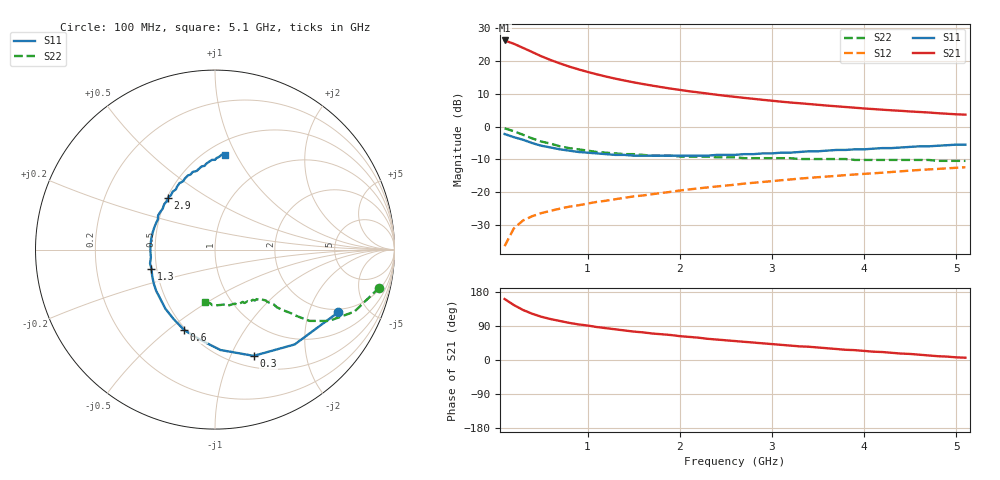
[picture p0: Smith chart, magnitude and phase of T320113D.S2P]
!AT-32011
!S PARAMETERS at Vce=2.7 V  Ic=7.5mA.  LAST UPDATED 01-05-95
# ghz s ma r 50
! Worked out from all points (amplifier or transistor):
!   51 points, 100 MHz to 5.1 GHz, reference 50 ohm
!   highest |S21| = 26.3 dB at 100 MHz (marker M1)
!   |S21| within 3 dB of that: start of sweep to 357.8 MHz
!   unconditionally stable (mu >= 1): 1.554 GHz to 4.921 GHz
!   at 900 MHz: K = 0.79, MSG = 20.7 dB, |S12| = -24.0 dB
!   at 2.6 GHz: K = 1.10, MAG = 11.5 dB, |S12| = -17.7 dB
!   at 5.1 GHz: K = 0.99, MSG = 8.0 dB, |S12| = -12.4 dB
!   S11 on the Smith chart (normalised r, x): 100 MHz: 1.84, -3.17; 300 MHz: 0.62, -1.23; 600 MHz: 0.49, -0.57; 1.3 GHz: 0.47, -0.12; 2.9 GHz: 0.51, +0.35; 5.1 GHz: 0.61, +0.90
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0.1  0.77 -27.0  20.59 161.0  0.015 76.0  0.94 -13.0
0.2  0.69 -50.0  18.33 145.0  0.028 67.0  0.85 -24.0
0.3  0.63 -70.0  15.87 132.0  0.037 60.0  0.75 -32.0
0.4  0.56 -87.0  13.7 122.0  0.043 55.0  0.66 -37.0
0.5  0.51 -99.0  11.8 114.0  0.048 53.0  0.59 -39.0
0.6  0.48 -111.0  10.35 108.0  0.052 52.0  0.55 -40.0
0.7  0.45 -121.0  9.2 103.0  0.056 51.0  0.5 -42.0
0.8  0.43 -130.0  8.24 98.0  0.06 51.0  0.47 -43.0
0.9  0.41 -138.0  7.47 94.0  0.063 51.0  0.45 -43.0
1  0.4 -145.0  6.82 91.0  0.067 51.0  0.43 -44.0
1.1  0.39 -151.0  6.27 87.0  0.071 51.0  0.41 -45.0
1.3  0.37 -163.0  5.39 81.0  0.078 52.0  0.39 -46.0
1.5  0.36 -173.0  4.73 75.0  0.086 52.0  0.38 -48.0
1.8  0.36 173.0  4 68.0  0.097 52.0  0.36 -51.0
2.1  0.36 160.0  3.46 61.0  0.11 51.0  0.35 -54.0
2.3  0.36 152.0  3.19 56.0  0.118 50.0  0.35 -57.0
2.6  0.37 142.0  2.84 50.0  0.13 49.0  0.34 -61.0
2.9  0.39 132.0  2.56 44.0  0.143 48.0  0.33 -64.0
3.5  0.42 115.0  2.15 33.0  0.169 44.0  0.32 -73.0
3.8  0.44 108.0  1.99 27.0  0.182 42.0  0.32 -77.0
4.3  0.47 97.0  1.77 19.0  0.203 39.0  0.31 -85.0
5.1  0.53 84.0  1.52 6.0  0.24 32.0  0.3 -101.0
